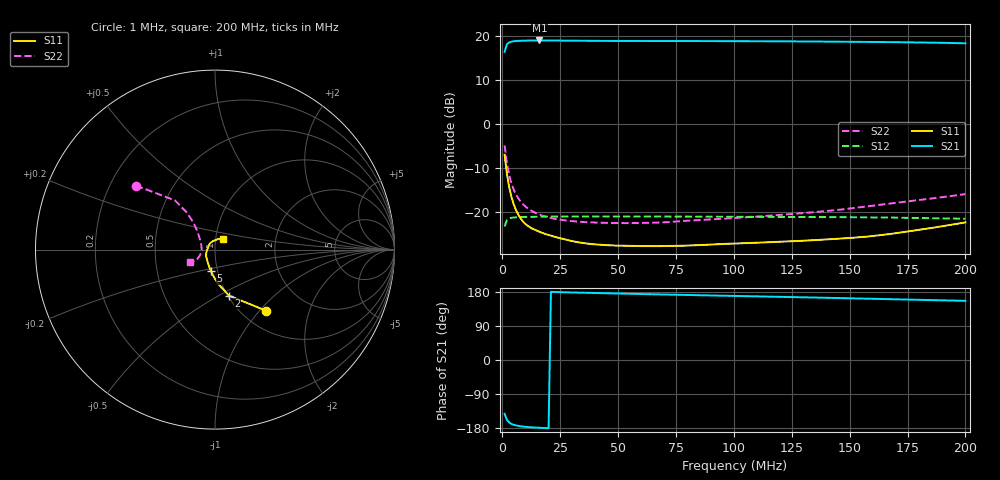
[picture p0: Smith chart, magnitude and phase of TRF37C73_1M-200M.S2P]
!Agilent Technologies,E5071B,JP1KK00322,A.09.10
!Date: Mon Jul 07 16:51:46 2014
!Data & Calibration Information:
!Freq		S11:SOLT2(ON)  S21:SOLT2(ON)  S12:SOLT2(ON)  S22:SOLT2(ON)
# Hz S dB R 50
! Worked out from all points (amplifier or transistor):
!   200 points, 1 MHz to 200 MHz, reference 50 ohm
!   highest |S21| = 18.9 dB at 16 MHz (marker M1)
!   |S21| within 3 dB of that: start of sweep to end of sweep
!   unconditionally stable (mu >= 1): start of sweep to end of sweep
!   at 34 MHz: K = 1.03, MAG = 18.9 dB, |S12| = -21.1 dB
!   at 101 MHz: K = 1.03, MAG = 18.8 dB, |S12| = -21.1 dB
!   at 200 MHz: K = 1.06, MAG = 18.5 dB, |S12| = -21.6 dB
!   S11 on the Smith chart (normalised r, x): 1 MHz: 1.28, -1.09; 2 MHz: 1.01, -0.56; 5 MHz: 0.93, -0.22; 200 MHz: 1.09, +0.13
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1000000  -7.04 -50.0  16.36 -141.9  -23.35 40.4  -4.94 141.0
2000000  -11.43 -73.0  18.08 -158.2  -21.89 22.9  -9.03 129.1
3000000  -14.50 -85.3  18.51 -165.1  -21.52 15.8  -11.74 127.3
4000000  -16.72 -94.1  18.67 -168.8  -21.38 12.0  -13.64 128.1
5000000  -18.41 -101.3  18.76 -171.2  -21.30 9.6  -15.06 130.0
6000000  -19.72 -107.6  18.81 -172.8  -21.25 8.0  -16.15 132.1
7000000  -20.75 -113.3  18.85 -174.0  -21.22 6.9  -17.02 134.4
8000000  -21.58 -118.5  18.87 -175.0  -21.20 5.9  -17.72 136.5
9000000  -22.25 -123.2  18.89 -175.7  -21.19 5.2  -18.31 138.6
1.2e7  -23.54 -135.5  18.93 -177.4  -21.15 3.6  -19.59 144.4
1.6e7  -24.55 -147.0  18.94 -178.8  -21.12 2.2  -20.64 150.7
2e7  -25.28 -155.2  18.93 -179.9  -21.11 1.3  -21.30 155.8
2.4e7  -25.88 -161.7  18.91 179.3  -21.10 0.6  -21.73 160.1
3.5e7  -27.12 -175.7  18.86 177.4  -21.09 -1.0  -22.34 169.2
4.4e7  -27.56 174.7  18.83 176.1  -21.09 -2.0  -22.51 174.8
6.8e7  -27.81 154.3  18.82 173.0  -21.10 -4.3  -22.45 -173.1
1.01e8  -27.22 132.1  18.78 169.0  -21.14 -7.2  -21.40 -162.9
1.34e8  -26.48 108.1  18.71 164.9  -21.20 -10.1  -20.12 -155.5
1.51e8  -25.93 94.3  18.65 162.7  -21.25 -11.6  -19.21 -152.3
1.67e8  -25.08 82.0  18.57 160.6  -21.32 -13.3  -18.17 -151.4
1.84e8  -23.79 67.8  18.45 158.3  -21.44 -15.0  -17.10 -151.8
2e8  -22.42 53.4  18.29 156.1  -21.59 -16.6  -15.99 -153.4
